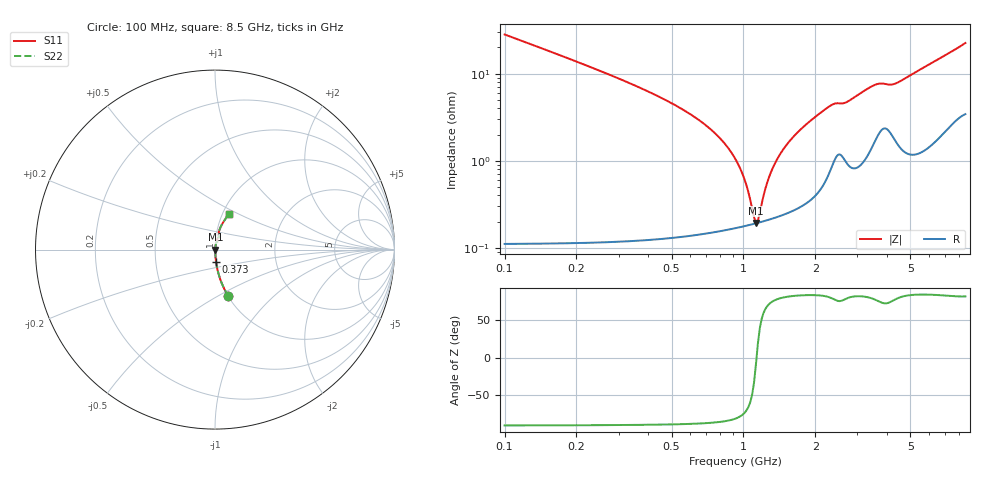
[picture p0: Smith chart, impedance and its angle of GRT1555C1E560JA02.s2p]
!Murata Part Number: GRT1555C1E560JA02
!These Parameters are Measured in Series Mode Connection
!Data Generated on Jun 19, 2026
!  o--ll--o
!Port1  Port2
!  o------o
!Operation Temp=25[degC], DC Bias Voltage=0[V]
!Freq. Start=100[MHz] Stop=9[GHz] 401[Steps]
# Hz S RI R 50
!Freq.(Hz) S11(Real) S11(Imag) S21(Real) S21(Imag) S12(Real) S12(Imag) S22(Real) S22(Imag)
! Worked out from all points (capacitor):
!   401 points, 100 MHz to 8.5 GHz, reference 50 ohm
!   read as one part in series: C = 56 pF near 142 MHz
!   lowest |Z| = 193 mohm at 1.129 GHz (marker M1)
!   series resonance near 1.135 GHz, so ESL is about 350 pH
!   S11 on the Smith chart (normalised r, x): 100 MHz: 1.00, -0.56; 373 MHz: 1.00, -0.14; 8.5 GHz: 1.07, +0.45
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1e8  0.0745 -0.2607  0.9255 0.2607  0.9255 0.2607  0.0745 -0.2607
2.26e8  0.0155 -0.1188  0.9845 0.1188  0.9845 0.1188  0.0155 -0.1188
3.73e8  0.00579 -0.0675  0.9942 0.0675  0.9942 0.0675  0.00579 -0.0675
7.3e8  0.002 -0.0228  0.998 0.0228  0.998 0.0228  0.002 -0.0228
8.77e8  0.0018 -0.013  0.9982 0.013  0.9982 0.013  0.0018 -0.013
9.82e8  0.00179 -0.00728  0.9982 0.00728  0.9982 0.00728  0.00179 -0.00728
1.024e9  0.00181 -0.00517  0.9982 0.00517  0.9982 0.00517  0.00181 -0.00517
1.087e9  0.00186 -0.00216  0.9981 0.00216  0.9981 0.00216  0.00186 -0.00216
1.129e9  0.00191 -0.000257  0.9981 0.000257  0.9981 0.000257  0.00191 -0.000257
1.171e9  0.00196 0.00158  0.998 -0.00158  0.998 -0.00158  0.00196 0.00158
1.255e9  0.00209 0.00509  0.9979 -0.00509  0.9979 -0.00509  0.00209 0.00509
1.318e9  0.00221 0.00759  0.9978 -0.00759  0.9978 -0.00759  0.00221 0.00759
1.402e9  0.0024 0.0108  0.9976 -0.0108  0.9976 -0.0108  0.0024 0.0108
1.507e9  0.00267 0.0146  0.9973 -0.0146  0.9973 -0.0146  0.00267 0.0146
1.78e9  0.00365 0.0241  0.9964 -0.0241  0.9964 -0.0241  0.00365 0.0241
2.2e9  0.00717 0.0381  0.9928 -0.0381  0.9928 -0.0381  0.00717 0.0381
2.914e9  0.0108 0.052  0.9892 -0.052  0.9892 -0.052  0.0108 0.052
3.586e9  0.0223 0.0702  0.9777 -0.0702  0.9777 -0.0702  0.0223 0.0702
4.3e9  0.0223 0.0716  0.9777 -0.0716  0.9777 -0.0716  0.0223 0.0716
5.707e9  0.026 0.1132  0.974 -0.1132  0.974 -0.1132  0.026 0.1132
7.114e9  0.0472 0.1543  0.9528 -0.1543  0.9528 -0.1543  0.0472 0.1543
8.5e9  0.0761 0.1991  0.9239 -0.1991  0.9239 -0.1991  0.0761 0.1991
